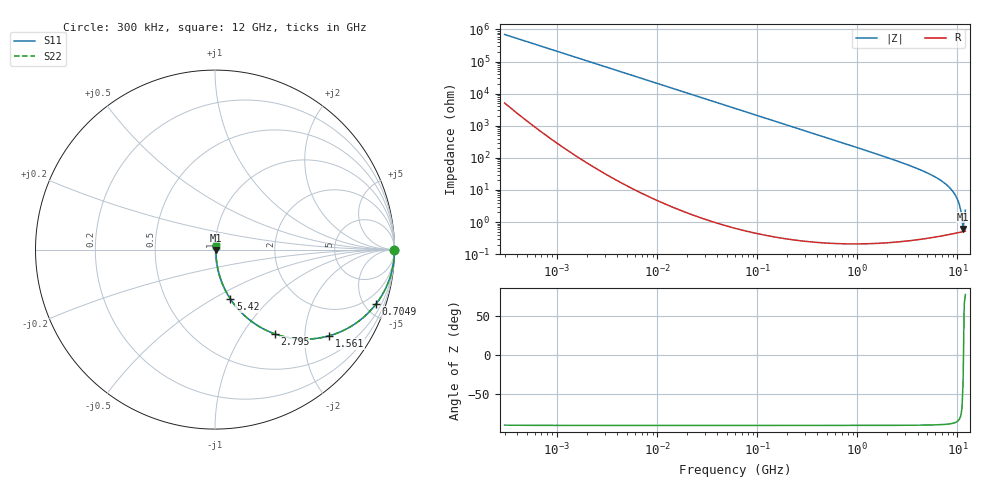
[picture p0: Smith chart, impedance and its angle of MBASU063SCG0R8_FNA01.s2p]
! MBASU063SCG0R8_FNA01  S-PARAMETER MODEL  ( Standard Model )
! Model Generated by TAIYO YUDEN Corporation (http://www.ty-top.com)
! Version 1.0
! TAIYO YUDEN Control No. 230609
! Copyright(c) 2023 TAIYO YUDEN CO.,LTD. All Rights Reserved.
! Product Description (link to TY-COMPAS)
! https://ds.yuden.co.jp/TYCOMPAS/or/detail?pn=MBASU063SCG0R8BFNA01&u=M
! Products Name : Multilayer Ceramic Capacitors
! Characteristics :
!  Capacitance : 0.8 [pF] , Rated Voltage : 50 [V] , TCC : CG / C0G
!  Case Size : 0.6 x 0.3 / 0.024 x 0.012 [mm/inch] , Thickness : 0.3 / 0.012 [mm/inch]
!  (Conditions: Temperature = 25 [degC] , DC Bias Voltage = 0 [V])
! External Node Assignments :
!  1  o---| |---o  2
! GND o---------o GND
! Frequency Range : 0.3MHz  -  12000MHz  [ 401 STEP ]
# MHZ S RI R 50
! Freq[MHz].  S11 Real  S11 Imag  S21 Real  S21 Imag  S12 Real  S12 Imag  S22 Real  S22 Imag
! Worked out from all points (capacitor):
!   401 points, 300 kHz to 12 GHz, reference 50 ohm
!   read as one part in series: C = 759 fF near 316.3 kHz
!   lowest |Z| = 614 mohm at 11.38 GHz (marker M1)
!   series resonance near 11.45 GHz, so ESL is about 250 pH
!   S11 on the Smith chart (normalised r, x): 300 kHz: open; 704.9 MHz: 1.00, -5.93; 1.561 GHz: 1.00, -2.64; 2.795 GHz: 1.00, -1.41; 5.42 GHz: 1.01, -0.60; 12 GHz: 1.01, +0.05
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0.3  1 -0.000143  1.07e-06 0.000143  1.07e-06 0.000143  1 -0.000143
1.769972  1 -0.000844  1.34e-06 0.000844  1.34e-06 0.000844  1 -0.000844
10.44266  1 -0.00498  2.59e-05 0.00498  2.59e-05 0.00498  1 -0.00498
60  0.9992 -0.0286  0.000823 0.0286  0.000823 0.0286  0.9992 -0.0286
164.1901  0.9939 -0.0778  0.00611 0.0778  0.00611 0.0778  0.9939 -0.0778
353.9943  0.9722 -0.1642  0.0278 0.1642  0.0278 0.1642  0.9722 -0.1642
704.9044  0.8977 -0.3027  0.1023 0.3027  0.1023 0.3027  0.8977 -0.3027
1048.836  0.797 -0.4017  0.203 0.4017  0.203 0.4017  0.797 -0.4017
1560.575  0.6349 -0.4806  0.3651 0.4806  0.3651 0.4806  0.6349 -0.4806
2088.533  0.4854 -0.4986  0.5146 0.4986  0.5146 0.4986  0.4854 -0.4986
2795.104  0.3331 -0.4696  0.6669 0.4696  0.6669 0.4696  0.3331 -0.4696
3944.255  0.1817 -0.3827  0.8183 0.3827  0.8183 0.3827  0.1817 -0.3827
5420.343  0.0854 -0.2741  0.9146 0.2741  0.9146 0.2741  0.0854 -0.2741
7254.098  0.0327 -0.1673  0.9673 0.1673  0.9673 0.1673  0.0327 -0.1673
8966.534  0.0124 -0.0895  0.9876 0.0895  0.9876 0.0895  0.0124 -0.0895
9968.853  0.00721 -0.051  0.9928 0.051  0.9928 0.051  0.00721 -0.051
10511.28  0.00577 -0.0317  0.9942 0.0317  0.9942 0.0317  0.00577 -0.0317
10793.46  0.00534 -0.0221  0.9947 0.0221  0.9947 0.0221  0.00534 -0.0221
11083.22  0.00509 -0.0125  0.9949 0.0125  0.9949 0.0125  0.00509 -0.0125
11380.75  0.00503 -0.00347  0.995 0.00347  0.995 0.00347  0.00503 -0.00347
11686.27  0.00524 0.011  0.9948 -0.011  0.9948 -0.011  0.00524 0.011
12000  0.00574 0.0227  0.9943 -0.0227  0.9943 -0.0227  0.00574 0.0227
